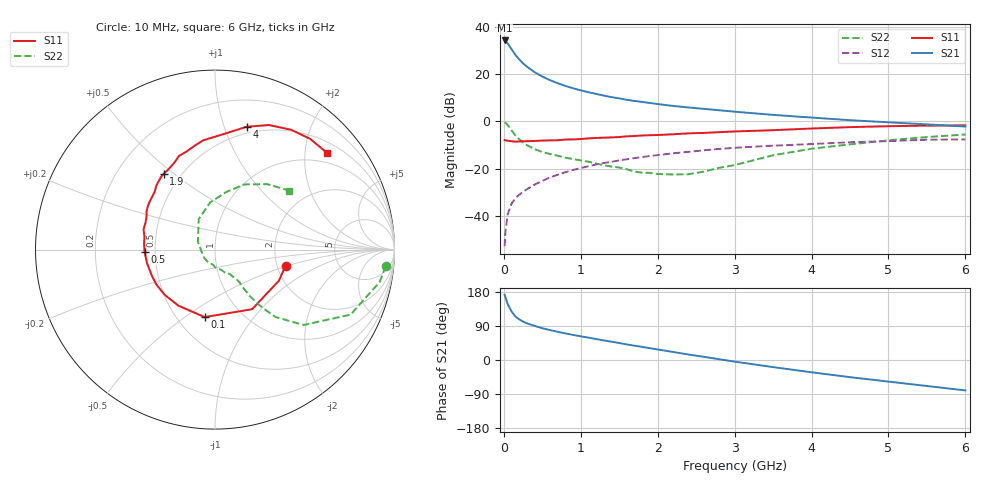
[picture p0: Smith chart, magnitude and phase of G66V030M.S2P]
! SIEMENS Small Signal Semiconductors
! BFG193
! Si NPN RF Bipolar Junction Transistor in SOT223
! VCE = 6 V  IC = 30 mA
! Common Emitter S-Parameters:  August  1996
# GHz  S  MA  R  50
!  f  S11  S21  S12  S22
! GHz  MAG  ANG  MAG  ANG  MAG  ANG  MAG  ANG
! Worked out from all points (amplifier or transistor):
!   36 points, 10 MHz to 6 GHz, reference 50 ohm
!   highest |S21| = 34.2 dB at 10 MHz (marker M1)
!   |S21| within 3 dB of that: start of sweep to 85.71 MHz
!   unconditionally stable (mu >= 1): 612.3 MHz to 2.392 GHz
!   at 250 MHz: K = 0.82, MSG = 27.2 dB, |S12| = -29.8 dB
!   at 1.4 GHz: K = 1.04, MAG = 12.4 dB, |S12| = -17.1 dB
!   at 6 GHz: K = 0.89, MSG = 2.7 dB, |S12| = -7.6 dB
!   S11 on the Smith chart (normalised r, x): 10 MHz: 2.23, -0.48; 100 MHz: 0.68, -0.60; 500 MHz: 0.44, -0.01; 1.9 GHz: 0.40, +0.46; 4 GHz: 0.44, +1.19; 6 GHz: 0.74, +2.48
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0.01  0.4035 -12.8  51.44 172.3  0.0023 89.2  0.9548 -5.5
0.02  0.3961 -25.9  50.33 166.0  0.0045 80.4  0.9353 -11.1
0.05  0.3912 -58.1  44.37 147.5  0.0109 71.5  0.838 -25.6
0.1  0.3805 -98.7  33.64 128.1  0.0182 66.1  0.6481 -40.4
0.15  0.3731 -123.2  25.53 114.9  0.0236 61.9  0.506 -48.0
0.2  0.377 -138.1  20.48 107.3  0.0282 63.4  0.4206 -50.7
0.25  0.3802 -149.2  16.86 101.2  0.0324 63.1  0.3548 -52.4
0.3  0.3808 -157.2  14.36 96.8  0.0368 64.5  0.3151 -53.3
0.4  0.3862 -168.7  10.99 90.1  0.0461 65.6  0.2583 -53.5
0.5  0.3927 -178.4  8.861 83.9  0.0552 64.9  0.2251 -53.2
0.6  0.3969 175.0  7.452 79.0  0.0653 64.4  0.2051 -54.1
0.8  0.4137 164.2  5.618 70.2  0.0844 62.1  0.1713 -57.5
1.1  0.4368 150.8  4.136 59.0  0.1126 57.5  0.1403 -66.4
1.4  0.4588 139.2  3.255 48.3  0.14 51.8  0.111 -78.9
1.9  0.5106 124.0  2.449 31.2  0.1853 41.5  0.0814 -115.8
2.2  0.5342 115.2  2.123 21.2  0.2111 34.7  0.0754 -145.1
2.8  0.5917 100.7  1.718 2.0  0.2617 21.0  0.1045 155.7
3.5  0.6516 84.4  1.373 -18.8  0.3069 4.1  0.1923 118.2
4  0.7065 75.6  1.205 -32.4  0.3318 -5.6  0.2642 95.8
4.5  0.7562 66.6  1.061 -45.3  0.3625 -15.7  0.3268 79.0
5.5  0.8133 49.3  0.864 -68.6  0.4094 -39.1  0.4661 51.5
6  0.8243 41.0  0.778 -80.3  0.4162 -52.5  0.5295 38.4
